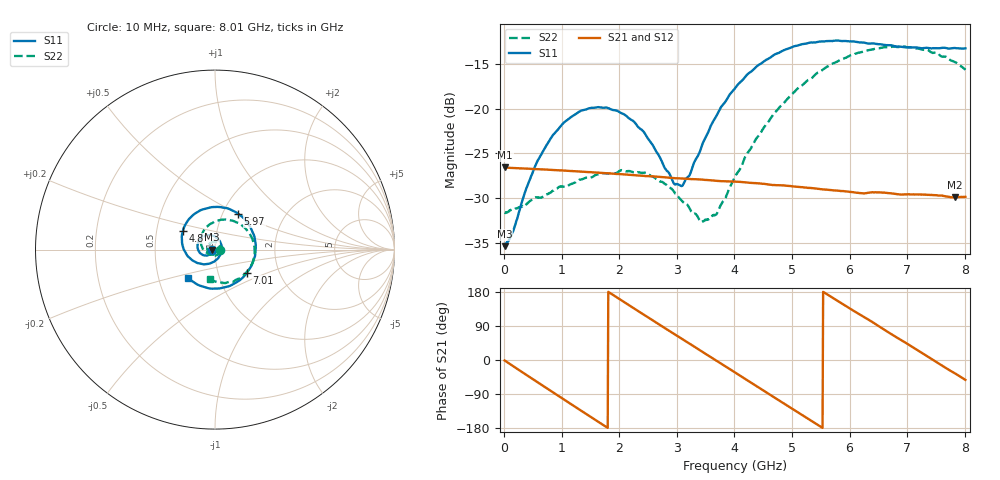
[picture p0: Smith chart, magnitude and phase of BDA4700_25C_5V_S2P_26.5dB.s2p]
!Agilent Technologies,E5071B,MY42404982,A.09.10
!Date: Mon Oct 20 13:39:51 2025
!Data & Calibration Information:
!Freq	S11:SOLT2(ON)	S21:SOLT2(ON)	S12:SOLT2(ON)	S22:SOLT2(ON)
# Hz S RI R 50
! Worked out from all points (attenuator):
!   801 points, 10 MHz to 8.01 GHz, reference 50 ohm
!   highest |S21| = -26.57 dB at 20 MHz (marker M1); lowest = -29.9 dB at 7.83 GHz (marker M2)
!   lowest |S11| = -35.4 dB at 10 MHz (marker M3), VSWR 1.03, Z = 48.3 - j0.102 ohm
!   |S11| at or under -10 dB: start of sweep to end of sweep
!   |S22| runs from -32.7 to -13.0 dB; largest |S21 - S12| = 0.00042
!   S11 on the Smith chart (normalised r, x): 10 MHz: 0.97, -0.00; 4.8 GHz: 0.68, +0.15; 5.97 GHz: 1.18, +0.50; 7.01 GHz: 1.37, -0.38; 8.01 GHz: 0.71, -0.23
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1e7  -0.017 -0.00106  0.0469 -0.000999  0.0469 -0.00105  0.0262 -0.00085
2e7  -0.0173 -0.00181  0.0469 -0.00175  0.0469 -0.0019  0.0261 -0.00108
1.5e8  -0.0181 -0.00951  0.0449 -0.0124  0.0449 -0.0124  0.0264 -0.00716
7e8  -0.0495 -0.0331  0.0153 -0.043  0.0153 -0.043  0.00598 -0.0321
1.03e9  -0.0798 -0.0222  -0.0103 -0.0439  -0.0103 -0.0439  -0.0164 -0.0327
1.35e9  -0.0973 0.00777  -0.0313 -0.0315  -0.0314 -0.0315  -0.0361 -0.0178
2.08e9  -0.0492 0.079  -0.0384 0.0192  -0.0384 0.0192  -0.0297 0.0336
2.68e9  0.0258 0.0488  -0.0037 0.0414  -0.00372 0.0413  0.0129 0.0375
2.95e9  0.0371 0.00889  0.0146 0.0382  0.0146 0.0382  0.0253 0.0232
3.1e9  0.0339 -0.0152  0.0236 0.0331  0.0235 0.0332  0.0281 0.0113
3.41e9  0.0044 -0.0586  0.0365 0.0169  0.0365 0.0169  0.0204 -0.0116
3.54e9  -0.0155 -0.0717  0.039 0.00849  0.039 0.00839  0.0129 -0.0204
3.7e9  -0.0463 -0.0802  0.0394 -0.0021  0.0395 -0.00223  -0.000768 -0.0261
4.01e9  -0.1103 -0.0686  0.0328 -0.0212  0.0329 -0.0212  -0.0323 -0.0258
4.8e9  -0.1782 0.1061  -0.0122 -0.0352  -0.0121 -0.0353  -0.0782 0.0673
5.35e9  -0.069 0.2237  -0.0342 -0.0111  -0.0342 -0.0111  -0.0156 0.1478
5.97e9  0.1292 0.1997  -0.026 0.0225  -0.0261 0.0225  0.1241 0.1502
6.68e9  0.2252 -0.0209  0.0102 0.0321  0.0102 0.0322  0.22 -0.000338
7.01e9  0.1771 -0.1305  0.0247 0.0222  0.0248 0.022  0.2013 -0.0885
7.45e9  0.0405 -0.2139  0.0329 -3.22e-05  0.0329 -0.000119  0.1129 -0.171
7.83e9  -0.097 -0.1955  0.026 -0.0185  0.026 -0.0186  0.0129 -0.1815
8.01e9  -0.1504 -0.1567  0.0196 -0.0255  0.0197 -0.0255  -0.0306 -0.1619
